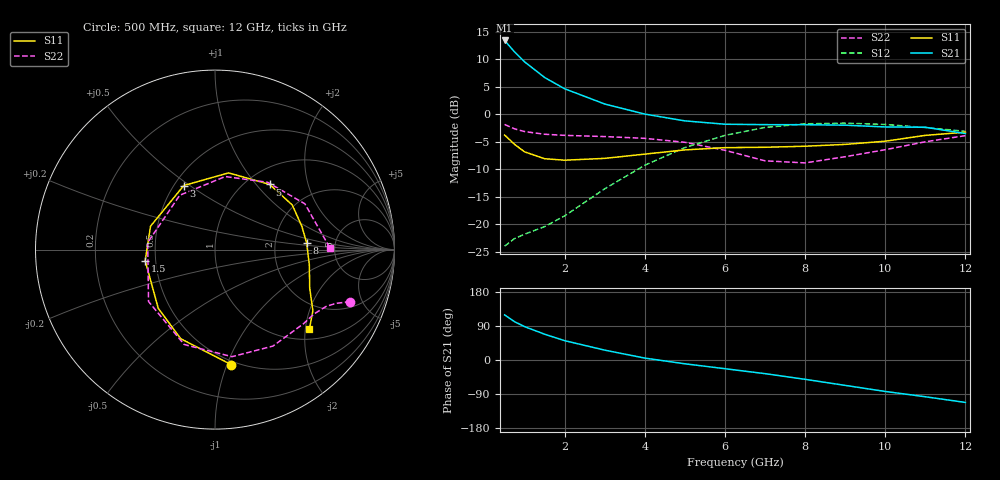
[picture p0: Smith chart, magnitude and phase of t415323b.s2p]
!AT-41532
!S-PARAMETERS at Vce=2.7V  Ic=2mA.  LAST UPDATED 05-29-98
# ghz s ma r 50
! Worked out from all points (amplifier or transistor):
!   15 points, 500 MHz to 12 GHz, reference 50 ohm
!   highest |S21| = 13.4 dB at 500 MHz (marker M1)
!   |S21| within 3 dB of that: start of sweep to 874.6 MHz
!   unconditionally stable (mu >= 1): 1.387 GHz to 2.414 GHz; 9.887 GHz to 10.1 GHz; 11.43 GHz to end of sweep
!   at 1 GHz: K = 0.83, MSG = 15.7 dB, |S12| = -21.8 dB
!   at 5 GHz: K = 0.79, MSG = 2.4 dB, |S12| = -6.1 dB
!   at 12 GHz: K = 1.01, MAG = -0.7 dB, |S12| = -3.1 dB
!   lowest NFmin = 1.20 dB at 900 MHz
!   S11 on the Smith chart (normalised r, x): 500 MHz: 0.47, -1.03; 1.5 GHz: 0.44, -0.06; 3 GHz: 0.56, +0.47; 5 GHz: 1.26, +1.18; 8 GHz: 3.07, +0.30; 12 GHz: 1.26, -2.11
0.5  0.647 -82.0  4.702 119.0  0.063 52.0  0.808 -21.0
0.75  0.532 -111.0  3.691 101.0  0.074 46.0  0.737 -24.0
1  0.455 -134.0  3 88.0  0.081 46.0  0.696 -27.0
1.5  0.394 -171.0  2.162 68.0  0.095 52.0  0.658 -33.0
2  0.382 160.0  1.707 51.0  0.119 59.0  0.643 -40.0
3  0.397 116.0  1.24 26.0  0.21 61.0  0.627 -59.0
4  0.434 80.0  1.004 5.0  0.344 50.0  0.604 -81.0
5  0.474 50.0  0.871 -10.0  0.498 32.0  0.556 -108.0
6  0.497 30.0  0.812 -23.0  0.643 11.0  0.47 -142.0
7  0.501 15.0  0.805 -36.0  0.759 -12.0  0.377 174.0
8  0.512 4.0  0.804 -51.0  0.819 -34.0  0.361 123.0
9  0.532 -9.0  0.796 -67.0  0.831 -55.0  0.411 82.0
10  0.569 -22.0  0.767 -83.0  0.808 -74.0  0.476 52.0
11  0.643 -32.0  0.762 -97.0  0.758 -93.0  0.562 27.0
12  0.687 -40.0  0.668 -112.0  0.7 -107.0  0.639 1.0
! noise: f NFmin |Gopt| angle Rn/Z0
0.9  1.2  0.35  100  0.17
1.8  1.6  0.48  -179  0.07
2  1.7  0.51  -165  0.07
2.5  1.9  0.6  -136  0.18
3  2.2  0.65  -112  0.42
3.5  2.5  0.7  -91  0.84
4  2.9  0.74  -74  1.44
